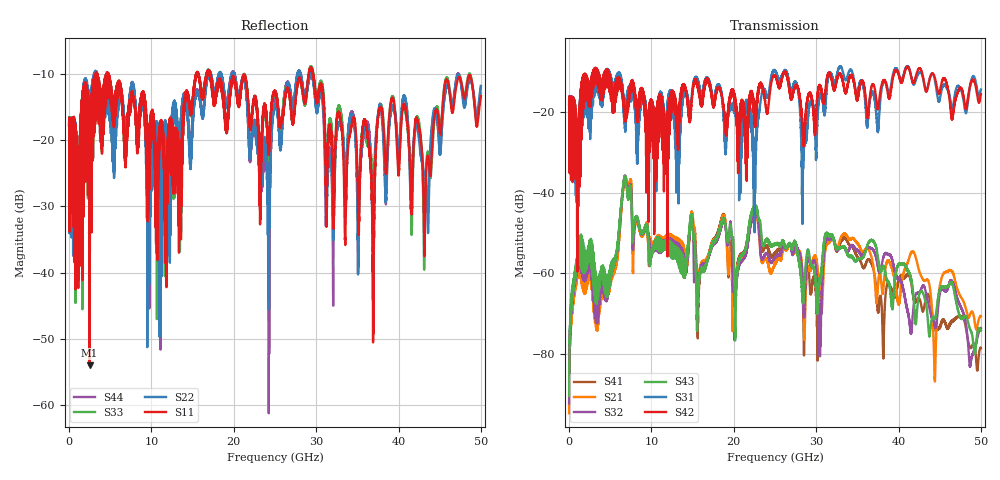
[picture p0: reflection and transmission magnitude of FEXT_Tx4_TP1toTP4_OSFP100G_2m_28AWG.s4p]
! Touchstone data
! Created: 27-Feb-2019 by IdEM 12 (12.1.0)
! COMMENTS
!  Created Wed Feb 27 12:03:36 2019
!  64 Port Network Data from SP1.SP block
!  freq  magS1_1  angS1_1  magS1_2  angS1_2  magS1_3  angS1_3  magS1_4  angS1_4
!  magS1_5  angS1_5  magS1_6  angS1_6  magS1_7  angS1_7  magS1_8  angS1_8
!  magS1_9  angS1_9  magS1_10  angS1_10  magS1_11  angS1_11  magS1_12  angS1_12
!  magS1_13  angS1_13  magS1_14  angS1_14  magS1_15  angS1_15  magS1_16  angS1_16
!  magS1_17  angS1_17  magS1_18  angS1_18  magS1_19  angS1_19  magS1_20  angS1_20
!  magS1_21  angS1_21  magS1_22  angS1_22  magS1_23  angS1_23  magS1_24  angS1_24
!  magS1_25  angS1_25  magS1_26  angS1_26  magS1_27  angS1_27  magS1_28  angS1_28
!  magS1_29  angS1_29  magS1_30  angS1_30  magS1_31  angS1_31  magS1_32  angS1_32
!  magS1_33  angS1_33  magS1_34  angS1_34  magS1_35  angS1_35  magS1_36  angS1_36
!  magS1_37  angS1_37  magS1_38  angS1_38  magS1_39  angS1_39  magS1_40  angS1_40
!  magS1_41  angS1_41  magS1_42  angS1_42  magS1_43  angS1_43  magS1_44  angS1_44
!  magS1_45  angS1_45  magS1_46  angS1_46  magS1_47  angS1_47  magS1_48  angS1_48
!  magS1_49  angS1_49  magS1_50  angS1_50  magS1_51  angS1_51  magS1_52  angS1_52
!  magS1_53  angS1_53  magS1_54  angS1_54  magS1_55  angS1_55  magS1_56  angS1_56
!  magS1_57  angS1_57  magS1_58  angS1_58  magS1_59  angS1_59  magS1_60  angS1_60
!  magS1_61  angS1_61  magS1_62  angS1_62  magS1_63  angS1_63  magS1_64  angS1_64
!  magS2_1  angS2_1  magS2_2  angS2_2  magS2_3  angS2_3  magS2_4  angS2_4
!  magS2_5  angS2_5  magS2_6  angS2_6  magS2_7  angS2_7  magS2_8  angS2_8
!  magS2_9  angS2_9  magS2_10  angS2_10  magS2_11  angS2_11  magS2_12  angS2_12
!  magS2_13  angS2_13  magS2_14  angS2_14  magS2_15  angS2_15  magS2_16  angS2_16
!  magS2_17  angS2_17  magS2_18  angS2_18  magS2_19  angS2_19  magS2_20  angS2_20
!  magS2_21  angS2_21  magS2_22  angS2_22  magS2_23  angS2_23  magS2_24  angS2_24
!  magS2_25  angS2_25  magS2_26  angS2_26  magS2_27  angS2_27  magS2_28  angS2_28
!  magS2_29  angS2_29  magS2_30  angS2_30  magS2_31  angS2_31  magS2_32  angS2_32
!  magS2_33  angS2_33  magS2_34  angS2_34  magS2_35  angS2_35  magS2_36  angS2_36
!  magS2_37  angS2_37  magS2_38  angS2_38  magS2_39  angS2_39  magS2_40  angS2_40
!  magS2_41  angS2_41  magS2_42  angS2_42  magS2_43  angS2_43  magS2_44  angS2_44
!  magS2_45  angS2_45  magS2_46  angS2_46  magS2_47  angS2_47  magS2_48  angS2_48
!  magS2_49  angS2_49  magS2_50  angS2_50  magS2_51  angS2_51  magS2_52  angS2_52
!  magS2_53  angS2_53  magS2_54  angS2_54  magS2_55  angS2_55  magS2_56  angS2_56
!  magS2_57  angS2_57  magS2_58  angS2_58  magS2_59  angS2_59  magS2_60  angS2_60
!  magS2_61  angS2_61  magS2_62  angS2_62  magS2_63  angS2_63  magS2_64  angS2_64
!  magS3_1  angS3_1  magS3_2  angS3_2  magS3_3  angS3_3  magS3_4  angS3_4
!  magS3_5  angS3_5  magS3_6  angS3_6  magS3_7  angS3_7  magS3_8  angS3_8
!  magS3_9  angS3_9  magS3_10  angS3_10  magS3_11  angS3_11  magS3_12  angS3_12
!  magS3_13  angS3_13  magS3_14  angS3_14  magS3_15  angS3_15  magS3_16  angS3_16
!  magS3_17  angS3_17  magS3_18  angS3_18  magS3_19  angS3_19  magS3_20  angS3_20
!  magS3_21  angS3_21  magS3_22  angS3_22  magS3_23  angS3_23  magS3_24  angS3_24
!  magS3_25  angS3_25  magS3_26  angS3_26  magS3_27  angS3_27  magS3_28  angS3_28
!  magS3_29  angS3_29  magS3_30  angS3_30  magS3_31  angS3_31  magS3_32  angS3_32
!  magS3_33  angS3_33  magS3_34  angS3_34  magS3_35  angS3_35  magS3_36  angS3_36
!  magS3_37  angS3_37  magS3_38  angS3_38  magS3_39  angS3_39  magS3_40  angS3_40
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# Hz S MA R 50
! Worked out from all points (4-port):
!   5000 points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, 10 MHz to 50 GHz, reference 50 ohm
!   strongest paths, dB at 10 MHz, 12.51 GHz, 25.01 GHz, 37.51 GHz, 50 GHz:
!     S42: -18.0, -18.0, -10.8, -19.1, -15.5
!     S31: -18.0, -16.4, -9.6, -24.1, -14.3
!     S43: -90.5, -53.9, -52.7, -56.2, -74.3
!     S32: -92.4, -52.7, -56.1, -58.6, -73.6
!     S21: -94.8, -51.3, -57.6, -63.0, -70.7
!     S41: -92.9, -52.4, -54.9, -69.7, -78.6
!   lowest |S11| = -54.1 dB at 2.49 GHz (marker M1), VSWR 1.00, Z = 49.8 + j0.0446 ohm
!   |S11| at or under -10 dB: 4.81 GHz to 15.41 GHz (10.6 GHz wide, 105 % of centre); 17.19 GHz to 29.09 GHz (11.9 GHz wide, 51.4 % of centre); 29.64 GHz to end of sweep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
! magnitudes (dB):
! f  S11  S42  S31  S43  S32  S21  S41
! 10 MHz  -17.7  -18.0  -18.0  -90.5  -92.4  -94.8  -92.9
! 2.49 GHz  -54.1  -17.0  -22.3  -56.1  -57.7  -59.3  -57.9
! 6.84 GHz  -21.0  -20.3  -19.4  -36.2  -36.0  -36.2  -36.2
! 15.65 GHz  -10.1  -14.1  -12.6  -65.0  -65.4  -62.5  -70.5
! 22.55 GHz  -13.9  -21.2  -42.2  -43.6  -45.1  -44.8  -43.8
! 24.88 GHz  -12.6  -10.8  -9.7  -53.0  -56.5  -58.4  -55.4
! 50 GHz  -13.3  -15.5  -14.3  -74.3  -73.6  -70.7  -78.6
